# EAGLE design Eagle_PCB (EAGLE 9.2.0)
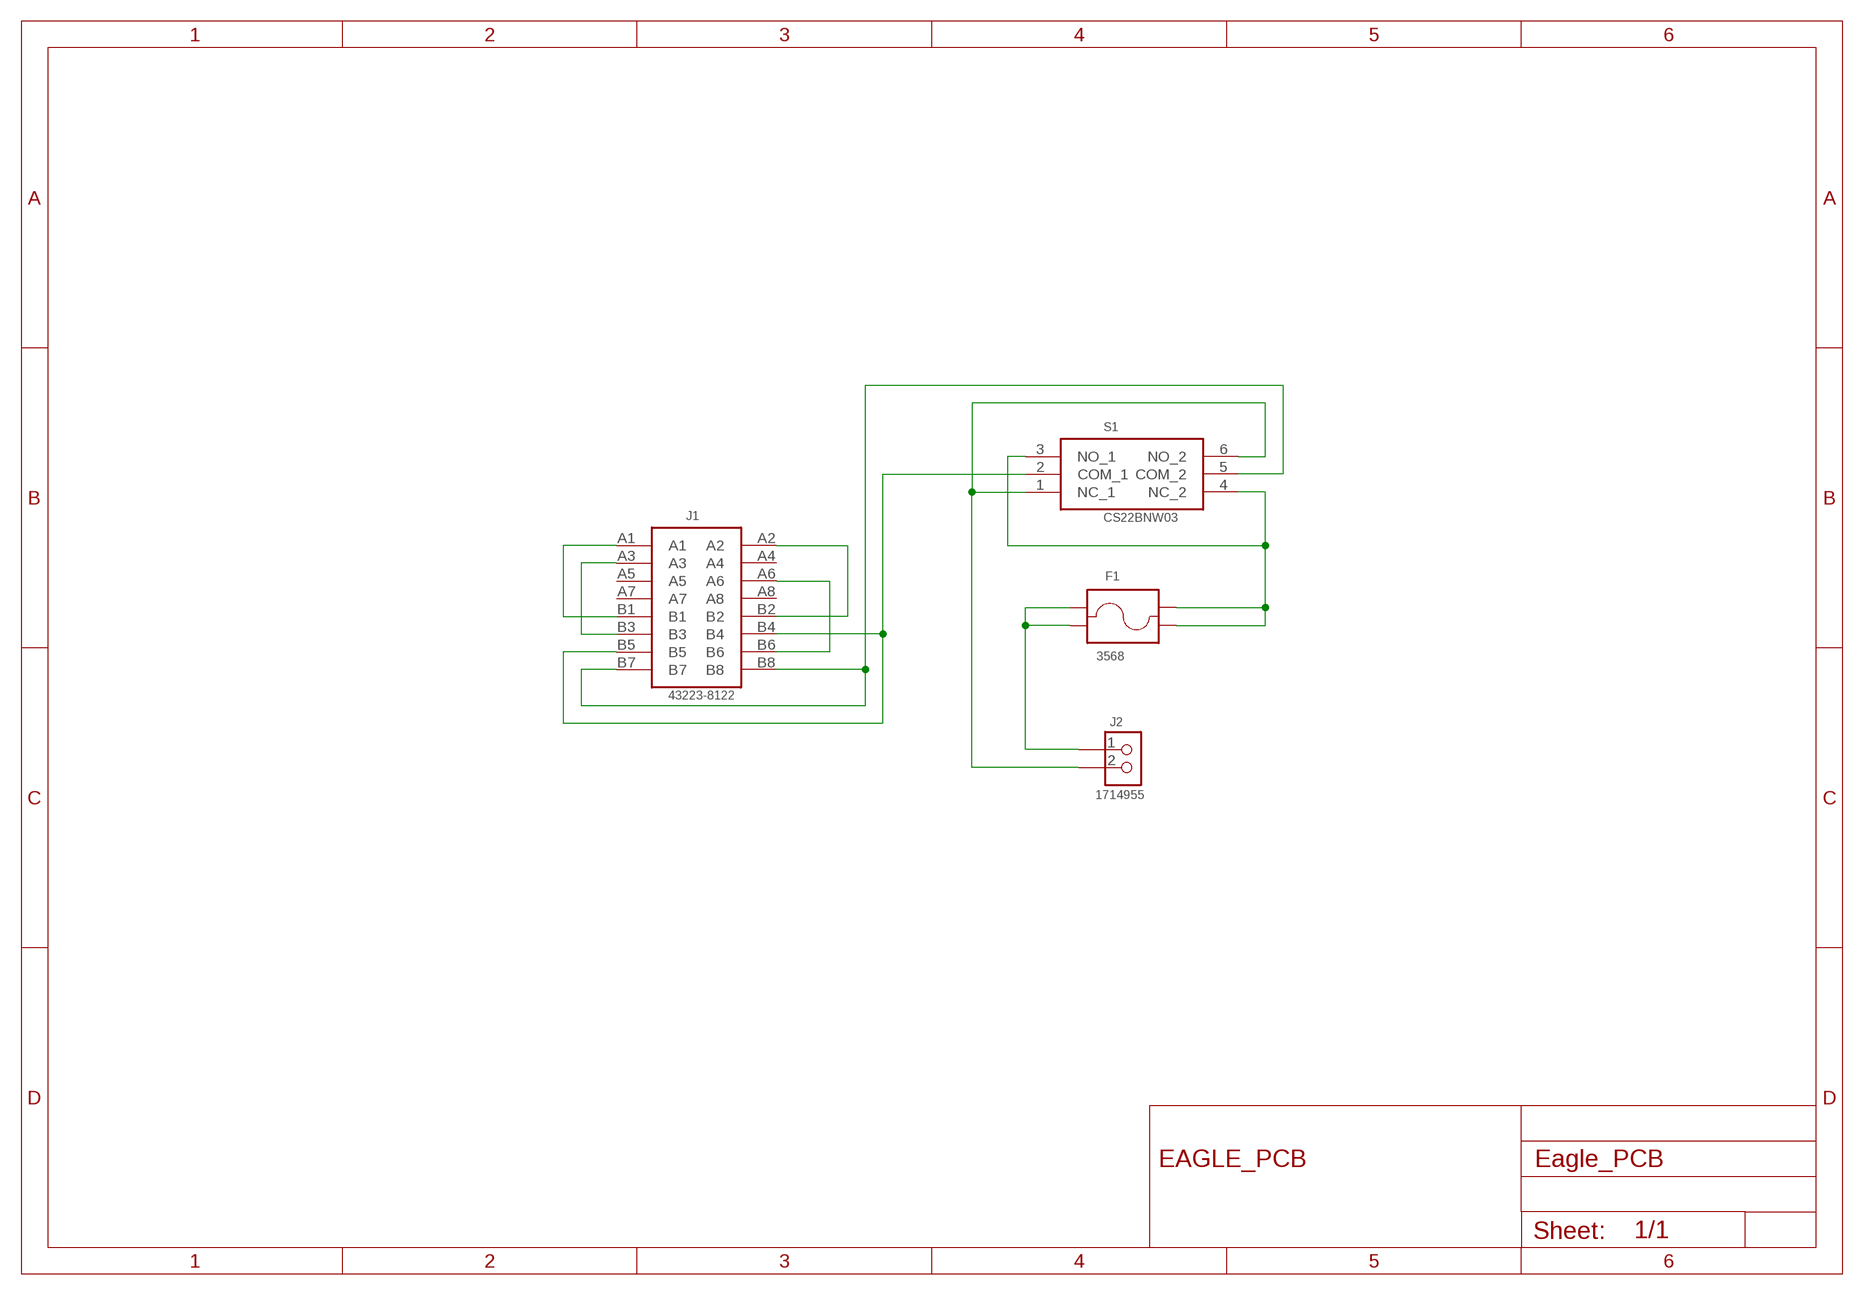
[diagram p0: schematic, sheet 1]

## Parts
F1  3568  [FUSE_3568]
J1  43223-8122  [43223-8122]
J2  1714955  [1714955]
S1  CS22BNW03  [CS22BNW03]

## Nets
N$1: J1.A1 J1.B1
N$2: J1.A3 J1.B3
N$3: J1.A2 J1.B2
N$4: J1.A6 J1.B6
N$5: J1.B7 J1.B8 S1.5(COM_2)
N$6: J1.B4 J1.B5 S1.2(COM_1)
N$7: J2.2 S1.1(NC_1) S1.6(NO_2)
N$8: F1.3 F1.4 S1.3(NO_1) S1.4(NC_2)
N$10: F1.1 F1.2 J2.1
Unconnected: J1.A4 J1.A5 J1.A7 J1.A8

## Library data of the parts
F1 = 3568:3568: Auto Fuse Holder; Mini; THM; 1 Fuse; 30Amp; Hi-Temp Nylon; UL94V-0; Brass/Tin Check prices; AVAILABILITY: In Stock; DESCRIPTION: THM-Vertical Entry Mini Auto Blade Fuse Holder; MF: Keystone Electronics; MP: 3568; PACKAGE: None; PRICE: None
J1 = 0432238122:43223-8122: PCB terminal block - MPT 0,5/ 2-2,54 - 1725656 Check prices; AVAILABILITY: In Stock; DESCRIPTION: CONN MOD JACK 8P8C R/A UNSHLD; MF: Molex; MP: 0432238122; PACKAGE: None; PRICE: None
J2 = Eagle_PCB:1714955: PCB terminal block - MPT 0,5/ 2-2,54 - 1725656 Check prices; AVAILABILITY: In Stock; DESCRIPTION: TERM BLK 2P SIDE ENT 6.35MM PCB; MF: Phoenix Contact; MP: 1714955; PACKAGE: None; PRICE: None
S1 = CS22BNW03:CS22BNW03: PCB terminal block - MPT 0,5/ 2-2,54 - 1725656 Check prices; AVAILABILITY: In Stock; DESCRIPTION: SWITCH SLIDE DPDT 3A 125V; MF: NKK Switches; MP: CS22BNW03; PACKAGE: None; PRICE: None

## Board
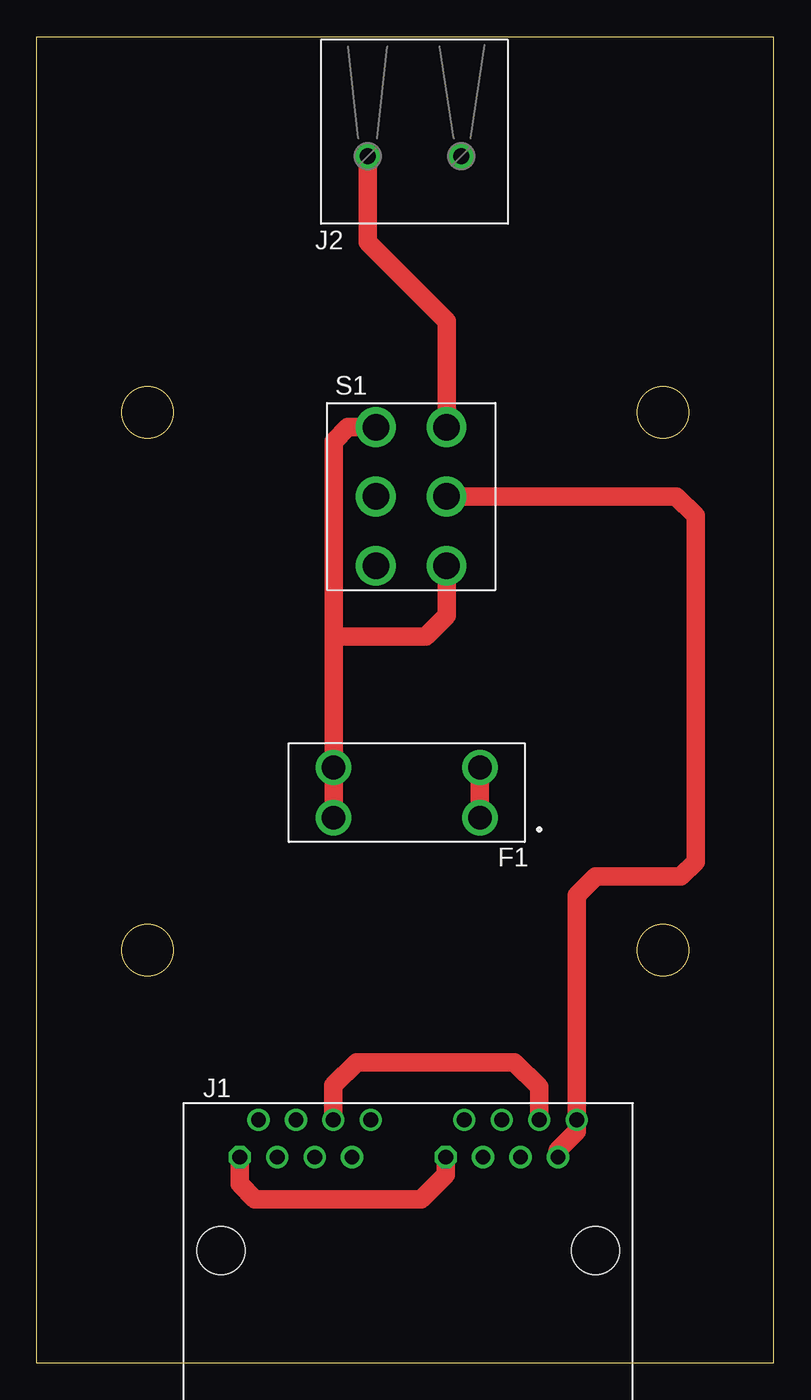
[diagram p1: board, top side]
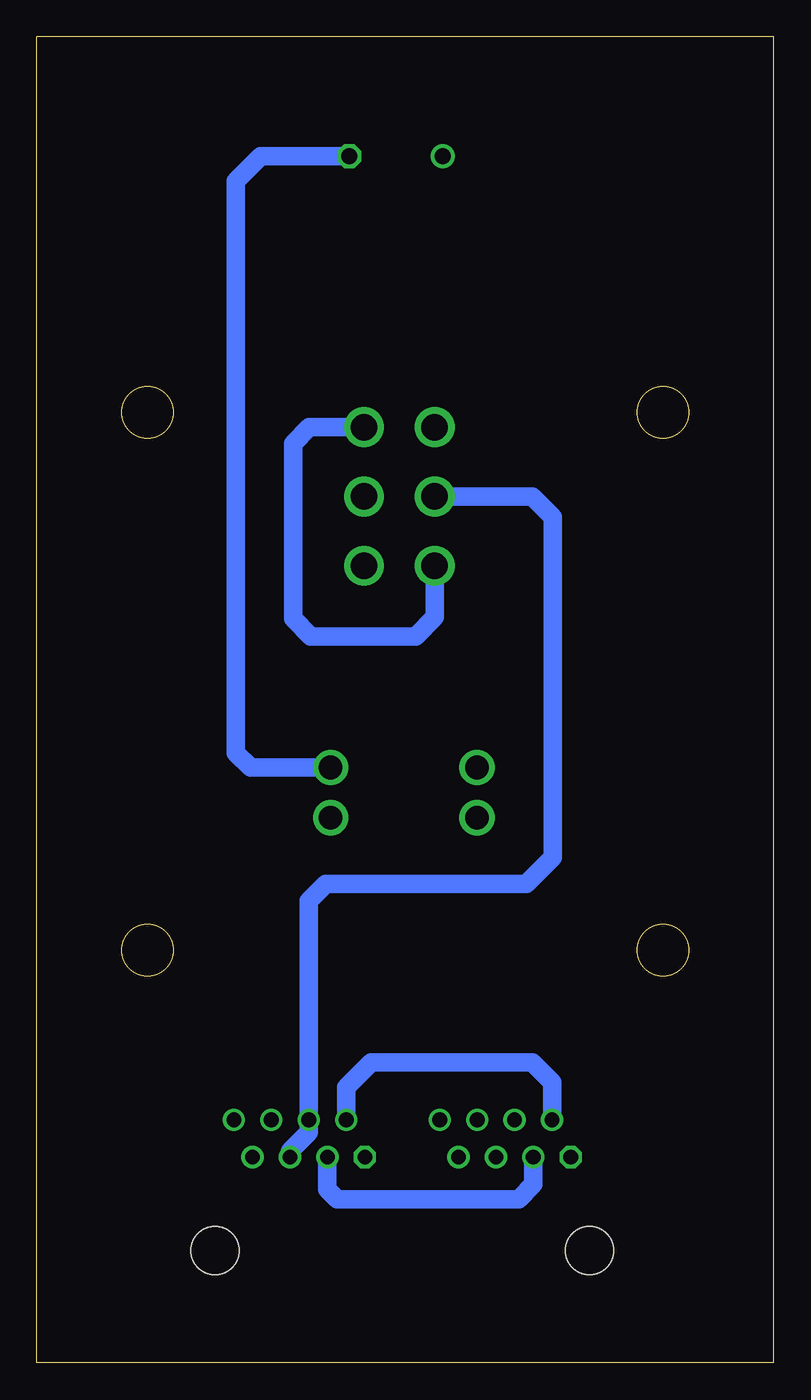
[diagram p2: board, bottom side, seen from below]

Size 50 x 90 mm. Coordinates in mm from the lower left corner, seen from the top.
Outline: 0,0 0,90 50,90 50,0 0,0
Outline: circle at 7.5,28 radius 1.75
Outline: circle at 42.5,28 radius 1.75
Outline: circle at 7.5,64.5 radius 1.75
Outline: circle at 42.5,64.5 radius 1.75
Copper layers (1+16): Top 0.035mm / dielectric 1.5mm / Bottom 0.035mm
Design rules "default *": minimum track width 8mil, minimum drill 0.35mm, track to track 8mil, track to pad 8mil, pad to pad 8mil, via to via 8mil, smd to smd 0mil, copper to edge 20mil, drill to drill 6mil, minimum pad ring 10mil, minimum via ring 8mil, stop-mask expansion 4mil, vias tented up to drill 0mil, thermal gap 10mil

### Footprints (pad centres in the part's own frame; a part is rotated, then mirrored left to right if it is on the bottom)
FUSE_3568 = drill 1.6: 1 -4.96,-1.7; 2 -4.96,1.7; 3 4.96,-1.7; 4 4.96,1.7
43223-8122 = drill 1 octagon: A1 1.27,6.35; B1 15.24,6.35 | drill 1: A2 2.54,8.89; A3 3.81,6.35; A4 5.08,8.89; A5 6.35,6.35; A6 7.62,8.89; A7 8.89,6.35; A8 10.16,8.89; B2 16.51,8.89; B3 17.78,6.35; B4 19.05,8.89; B5 20.32,6.35; B6 21.59,8.89; B7 22.86,6.35; B8 24.13,8.89 | hole 3.25: 0,0; 25.4,0
1714955 = drill 1.1 octagon: 1 0,0 | drill 1.1: 2 6.35,0
CS22BNW03 = drill 1.8: 1 -2.4,-4.7; 2 -2.4,0; 3 -2.4,4.7; 4 2.4,-4.7; 5 2.4,0; 6 2.4,4.7

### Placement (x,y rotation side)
F1  25.1,38.7 180 top
J1  12.5,7.6 0 top
J2  28.8,81.9 180 top
S1  25.4,58.8 0 top

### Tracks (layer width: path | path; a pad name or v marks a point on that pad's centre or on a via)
N$1
  Top 1.27: J1.A1 13.77,12.13 14.8,11.1 26.1,11.1 27.74,12.74 J1.B1
N$2
  Bottom 1.27: J1.A3 16.31,12.09 17.3,11.1 29.6,11.1 30.28,11.78 J1.B3
N$3
  Bottom 1.27: J1.A2 15.04,19.04 16.4,20.4 27.3,20.4 29.01,18.69 J1.B2
N$4
  Top 1.27: J1.A6 20.12,18.82 21.7,20.4 32.4,20.4 34.09,18.71 J1.B6
N$5
  Top 1.27: J1.B7 35.36,14.42 36.63,15.69 J1.B8 36.63,31.7 37.93,33 43.7,33 44.7,34 44.7,57.5 43.4,58.8 S1.5
N$6
  Bottom 1.27: S1.2 16.4,58.8 15,57.4 15,34.3 16.8,32.5 30.41,32.5 31.55,31.36 J1.B4 31.55,15.65 32.82,14.38 J1.B5
N$7
  Top 1.27: S1.6 27.8,70.7 22.45,76.05 J2.2
  Bottom 1.27: S1.6 31.5,63.5 32.6,62.4 32.6,50.5 31.4,49.3 24.3,49.3 23,50.6 S1.1
N$8
  Top 1.27: F1.4 F1.3 20.14,49 | S1.3 21.1,63.5 20.14,62.54 20.14,49 | S1.4 27.8,50.7 26.4,49.3 20.44,49.3 20.14,49
N$10
  Top 1.27: F1.2 F1.1
  Bottom 1.27: F1.1 35.5,40.4 36.5,41.4 36.5,80.2 34.8,81.9 J2.1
